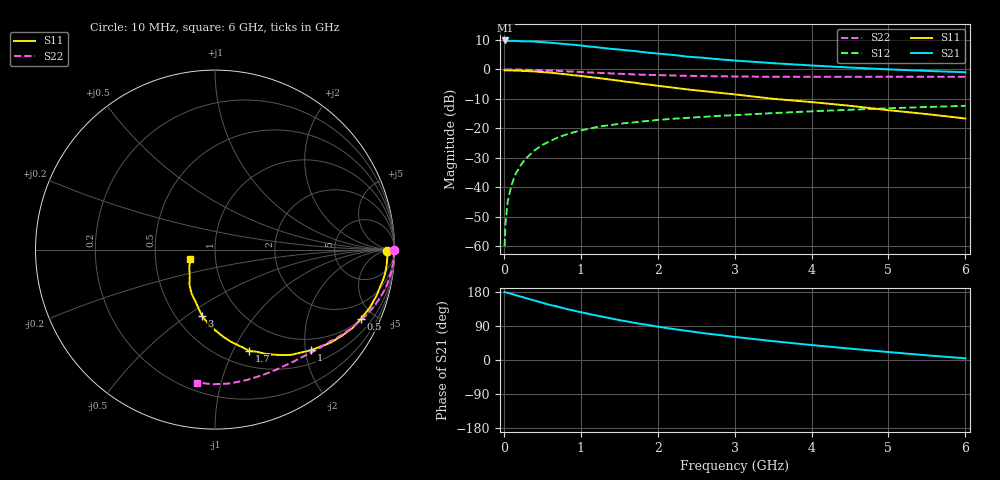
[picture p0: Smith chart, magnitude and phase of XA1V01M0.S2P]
! SIEMENS Discrete & RF Semiconductors
! BFY180
! Si NPN RF Bipolar Junction Transistor in MICRO-X
! VCE = 1 V  IC = 1 mA
! Common Emitter S-Parameters:  May  1997
# GHz  S  MA  R  50
!  f  S11  S21  S12  S22
! GHz  MAG  ANG  MAG  ANG  MAG  ANG  MAG  ANG
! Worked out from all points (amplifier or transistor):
!   36 points, 10 MHz to 6 GHz, reference 50 ohm
!   highest |S21| = 9.8 dB at 20 MHz (marker M1)
!   |S21| within 3 dB of that: start of sweep to 1.464 GHz
!   unconditionally stable (mu >= 1): 3.071 GHz to end of sweep
!   at 250 MHz: K = 0.09, MSG = 20.5 dB, |S12| = -31.4 dB
!   at 1.4 GHz: K = 0.59, MSG = 12.9 dB, |S12| = -18.9 dB
!   at 6 GHz: K = 1.12, MAG = 3.6 dB, |S12| = -12.4 dB
!   S11 on the Smith chart (normalised r, x): 10 MHz: 47, -8; 500 MHz: 1.04, -4.21; 1 GHz: 0.75, -2.11; 1.7 GHz: 0.66, -1.16; 3 GHz: 0.67, -0.57; 6 GHz: 0.75, -0.08
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0.01  0.9596 -0.4  3.026 179.6  0.001 97.8  0.997 -0.2
0.02  0.9598 -1.0  3.098 178.8  0.0023 91.1  0.9999 -0.5
0.05  0.9609 -2.4  3.053 177.2  0.0057 88.2  0.9966 -1.4
0.1  0.9604 -5.1  3.046 174.5  0.0109 86.6  0.9965 -2.9
0.15  0.9572 -7.9  3.052 171.4  0.0165 85.1  0.9964 -4.4
0.3  0.9378 -15.2  3.002 162.5  0.0319 79.5  0.9851 -8.7
0.4  0.9224 -20.3  2.966 156.8  0.0423 75.7  0.9788 -11.4
0.5  0.9 -25.3  2.905 151.1  0.0522 72.2  0.9681 -14.1
0.6  0.8821 -29.7  2.837 145.3  0.0607 69.2  0.9559 -16.6
0.8  0.8271 -38.8  2.687 135.3  0.0774 63.4  0.9296 -21.5
1  0.7745 -46.4  2.541 126.2  0.0918 58.1  0.9027 -25.9
1.1  0.746 -50.3  2.453 121.9  0.098 55.5  0.8891 -27.9
1.4  0.667 -61.3  2.23 109.4  0.1141 49.3  0.8527 -33.6
1.7  0.5951 -71.4  2.049 98.1  0.1266 44.5  0.8201 -38.5
2  0.5272 -79.4  1.858 88.0  0.1388 40.4  0.8013 -43.1
2.2  0.4902 -84.3  1.758 81.8  0.1453 37.8  0.7885 -46.1
2.6  0.4275 -93.3  1.572 70.7  0.1565 34.0  0.7692 -51.4
3  0.3766 -101.1  1.415 60.9  0.1673 30.2  0.7579 -56.8
3.5  0.3171 -109.2  1.275 49.8  0.1813 26.5  0.7507 -63.2
4.5  0.2413 -126.2  1.075 30.0  0.2066 18.4  0.7478 -76.6
5.5  0.1743 -145.3  0.942 12.3  0.2303 10.2  0.7502 -90.7
6  0.1467 -159.4  0.895 4.5  0.2404 5.8  0.7475 -97.8
